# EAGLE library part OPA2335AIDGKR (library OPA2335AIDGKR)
Check availability
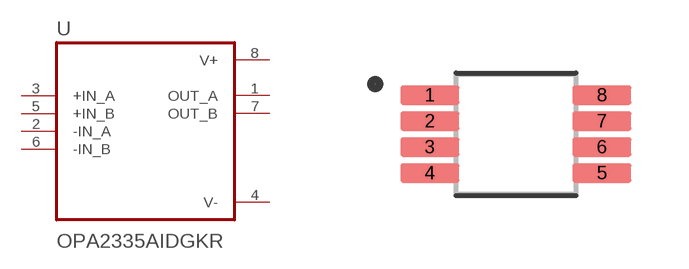
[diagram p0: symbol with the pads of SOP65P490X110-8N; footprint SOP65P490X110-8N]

Designator prefix U

## OPA2335AIDGKR (Availability: In Stock; Description: Dual 0.05uV/C max, single-supply CMOS operational amplifier; MF: Texas Instruments; MP: OPA2335AIDGKR; Package: VSSOP-8 Texas Instruments; Price: None; Purchase-URL: https://pricing.snapeda.com/search/part/OPA2335AIDGKR/?ref=eda)  [SOP65P490X110-8N]
1  OUT_A  out
2  -IN_A  in
3  +IN_A  in
4  V-  pwr
5  +IN_B  in
6  -IN_B  in
7  OUT_B  out
8  V+  pwr

## Footprint SOP65P490X110-8N (pad centres in mm)
smd 1.47 x 0.48: 1 -2.15,0.975; 2 -2.15,0.325; 3 -2.15,-0.325; 4 -2.15,-0.975; 5 2.15,-0.975; 6 2.15,-0.325; 7 2.15,0.325; 8 2.15,0.975

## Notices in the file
This work is licensed under a Creative Commons Attribution-ShareAlike 4.0 International License (CC BY-SA) with Design Exception 1.0
